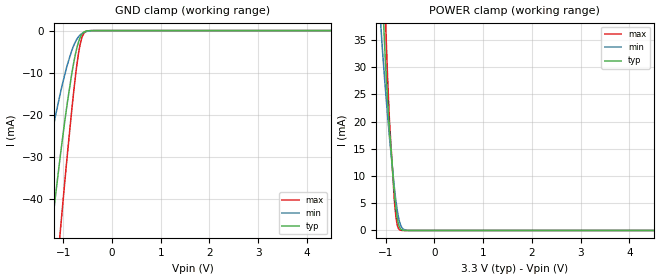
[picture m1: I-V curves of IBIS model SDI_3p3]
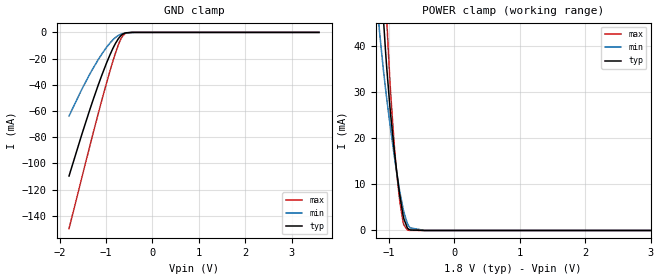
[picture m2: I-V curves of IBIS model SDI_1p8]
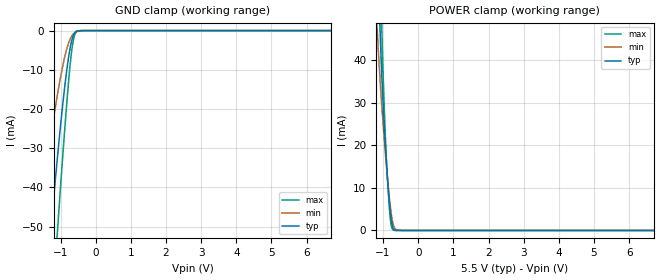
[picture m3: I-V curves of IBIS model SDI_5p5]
|Texas Instruments Incorporated
| 12-Bit Analog Monitor and Control Solution with
| Multichannel ADC, Bipolar DACs adn Temperature Sensors
| Marketing part#   Digital Voltage Range   Package-type   #pins
| AMC7832   1.8V - 5.5V   PQFP   64
[IBIS Ver]   4.1
[File name]   amc7832.ibs
[File Rev]   1.0
[Date]   07/17/2013
[Source]
| Texas Instruments Incorporated.
| Analog-eLab Design Center, HPA
| 12500 TI Blvd
| Dallas, TX -75243
[Notes]   Revision History:
| Rev 1.0: 07/17/2013
| - Initial version of the model
| - Model generated from simulations in TISPICE
| - C_comp although listed in numerical order of value are
|   obtained from varying PVT conditions. For PVT conditions for
|   each specific value refer the buffer description under
|   respective [Model]. IBIS model user is responsible for using
|   appropriate C_comp to simulate for Signal Integrity.
| - Warnings regarding combined Non-monotonicity of various models have been
|   reviewd and considered minor and can be ignored.
| - Model names with a trailing _1p8 contains the model for
|   1.8V operation.Model names with a trailing _3p3 contains the model
|   for 3.3V operation.Model names with a trailing _5p5 contains the model
|   for 5.5V operation.
| - Please note GPIO model is broken into two models depending on its mode
|   of operation (output or input).
[Disclaimer]
| This model is designed as an aid for customers of Texas Instruments.
| TI and its licensors and suppliers make no warranties, either expressed
| or implied, with respect to this  model, including the warranties of
| merchantability or fitness for a particular purpose. The model is
| provided solely on an "as is" basis. The entire risk as to its quality
| and performance is with the customer.
[Copyright]
 (C) Copyright 2013 Texas Instruments Incorporated.All rights reserved.
|   Device
[Component]   TPS51219
[Manufacturer]   TI
[Package]
| PQFP   64
|   typ   min   max
R_pkg   0.116   0.060   0.158
L_pkg   3.087nH   2.446nH   3.790nH
C_pkg   0.477pF   0.441pF   0.609pF
[Pin]  signal_name   model_name   R_pin   L_pin   C_pin
1   DGND   GND   0.07464   2.98837nH   0.48958pF
2   DVDD   POWER   0.13169   3.27499nH   0.48108pF
3   IOVDD   POWER   0.12816   3.19692nH   0.47536pF
4   RESETB   SDI   0.12615   3.14632nH   0.4667pF
5   SDO   SDO   0.12893   3.19318nH   0.46127pF
6   SDI   SDI   0.12666   3.13713nH   0.45672pF
7   SCLK   SDI   0.12544   3.10425nH   0.45279pF
8   CSB   SDI   0.12462   3.08462nH   0.44445pF
9   GPIO0/ALARMINB   GPIO   0.12195   3.03196nH   0.44282pF
10   GPIO1/ALARMOUTB   GPIO   0.12154   3.02759nH   0.45119pF
11   GPIO2/ADCTRIGB   GPIO   0.12196   3.04505nH   0.45655pF
12   GPIO3/DAVB   GPIO   0.12318   3.07964nH   0.46318pF
13   GPIO4   GPIO   0.12516   3.12641nH   0.47241pF
14   GPIO5   GPIO   0.12831   3.19935nH   0.47997pF
15   GPIO6   GPIO   0.13267   3.29462nH   0.48661pF
16   GPIO7   GPIO   0.13863   3.43954nH   0.44655pF
17   AVEE   GND   0.07231   2.94556nH   0.4856pF
18   DAC_A11   NC   0.13114   3.27314nH   0.48478pF
19   DAC_A10   NC   0.12565   3.15687nH   0.47686pF
20   AVSS_A   NC   0.06539   2.59229nH   0.51673pF
21   VRANGE_A   NC   0.12005   3.02694nH   0.45909pF
22   DAC_A9   NC   0.11967   3.00768nH   0.45569pF
23   AGND1   GND   0.06348   2.50448nH   0.4998pF
24   DAC_A8   NC   0.11877   2.97614nH   0.44498pF
25   AVCC_AB   POWER   0.06352   2.44605nH   0.49873pF
26   VRANGE_B   NC   0.1175   2.95523nH   0.4486pF
27   DAC_B7   NC   0.12033   3.02069nH   0.45459pF
28   AVSS_B   GND   0.06484   2.56764nH   0.51127pF
29   DAC_B6   NC   0.12376   3.1084nH   0.4693pF
30   REF_OUT1   NC   0.12489   3.14114nH   0.47142pF
31   AVDD1   POWER   0.12943   3.23893nH   0.48258pF
32   REF_CMP   NC   0.07299   2.86238nH   0.49781pF
33   AGND2   GND   0.06024   3.09923nH   0.58549pF
34   AVDD2   POWER   0.08563   3.23091nH   0.60933pF
35   ADC_11   NC   0.15758   3.7897nH   0.52144pF
36   ADC_10   NC   0.14845   3.5965nH   0.5063pF
37   ADC_9   NC   0.14092   3.43726nH   0.49064pF
38   ADC_8   NC   0.13472   3.30228nH   0.47781pF
39   ADC_7   NC   0.12993   3.19697nH   0.46698pF
40   ADC_6   NC   0.12655   3.12518nH   0.455pF
41   LV_ADC16   NC   0.12409   3.07578nH   0.44888pF
42   LV_ADC15   NC   0.1236   3.07045nH   0.45215pF
43   LV_ADC14   NC   0.12381   3.08372nH   0.4563pF
44   LV_ADC13   NC   0.12473   3.11302nH   0.46145pF
45   LV_ADC_12   NC   0.1263   3.15208nH   0.46839pF
46   ADC_5   NC   0.12888   3.2135nH   0.47766pF
47   ADC_4   NC   0.13439   3.32975nH   0.48914pF
48   ADC_3   NC   0.14231   3.51158nH   0.45064pF
49   ADC_2   NC   0.13353   3.33493nH   0.44139pF
50   ADC_1   NC   0.12597   3.15979nH   0.47985pF
51   ADC_0   NC   0.12099   3.05316nH   0.46759pF
52   DAC_C0   NC   0.12205   3.06323nH   0.46543pF
53   AVSS_C   GND   0.06421   2.5389nH   0.50917pF
54   DAC_C1   NC   0.11943   2.99201nH   0.45501pF
55   VRANGE_C   NC   0.11829   2.9599nH   0.4497pF
56   REF_OUT2   NC   0.11893   2.96848nH   0.44539pF
57   AVCC_CD   POWER   0.06422   2.46561nH   0.5006pF
58   DAC_D2   NC   0.12085   3.01039nH   0.45506pF
59   AGND3   GND   0.06535   2.574nH   0.51014pF
60   DAC_D3   NC   0.12454   3.10478nH   0.46658pF
61   VRANGE_D   NC   0.12732   3.16823nH   0.47473pF
62   AVSS_D   GND   0.06959   2.7448nH   0.53356pF
63   DAC_D4   NC   0.13598   3.35887nH   0.49213pF
64   DAC_D5   NC   0.14445   3.55251nH   0.45417pF
|   Model Selectors
[Model Selector]  SDI
SDI_3p3   input buffer with 3.3V operation
SDI_1p8   input buffer with 1.8V operation
SDI_5p5   input buffer with 5.5V operation
[Model Selector]  SDO
SDO_3p3   output buffer with 3.3V operation
SDO_1p8   output buffer with 1.8V operation
SDO_5p5   output buffer with 5.5V operation
[Model Selector]  GPIO
GPIO_OUT_3p3   ouput mode with 3.3V operation
GPIO_OUT_1p8   ouput mode with 1.8V operation
GPIO_OUT_5p5   ouput mode with 5.5V operation
GPIO_IN_3p3   input mode with 3.3V operation
GPIO_IN_1p8   input mode with 1.8V operation
GPIO_IN_5p5   input mode with 5.5V operation
| Models and submodels in the file (12): SDI_3p3 (Input), SDI_1p8 (Input), SDI_5p5 (Input), SDO_5p5 (Output), SDO_3p3 (Output), SDO_1p8 (Output), GPIO_OUT_5p5 (Output), GPIO_OUT_3p3 (Output), GPIO_OUT_1p8 (Output), GPIO_IN_5p5 (Input), GPIO_IN_3p3 (Input), GPIO_IN_1p8 (Input)
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|   Model
[Model]   SDI_3p3
Model_type   Input
Vinl = 0.99
Vinh = 2.31
|   typ   min   max
C_comp   1pF   1pF   1pF
[Voltage Range]   3.3   3.29   3.31
[Temperature Range]   27   125   -40
[Power Clamp Reference]   3.3   3.29   3.31
[GND Clamp Reference]   -0   -0   -0
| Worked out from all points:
|   GND clamp passes 1 mA (typ) near -0.62 V on its own axis
|   POWER clamp passes 1 mA (typ) near -0.73 V on its own axis
[GND Clamp]
|   Voltage   I(typ)   I(min)   I(max)
-3.3V     -293.4mA   -195.7mA   -362.8mA
-1.607V   -87.33mA   -49.37mA   -122.6mA
-1.498V   -75.05mA   -41.65mA   -107.3mA
-1.241V   -47.39mA   -24.95mA   -71.62mA
-1.063V   -29.88mA   -14.98mA   -47.85mA
-914.1mV  -16.91mA   -8.021mA   -29.15mA
-825mV    -10.21mA   -4.72mA    -18.75mA
-735.9mV  -4.854mA   -2.34mA    -9.493mA
-646.8mV  -1.481mA   -966.8uA   -2.922mA
-597.3mV  -576.8uA   -553.5uA   -1.078mA
-547.8mV  -186.8uA   -301.2uA   -307.2uA
6.59V     0A         0A         0A
[POWER Clamp]
|   Voltage   I(typ)   I(min)   I(max)
-3.3V     807.6mA    663.4mA    932mA
-1.122V   56.01mA    40.38mA    75.28mA
-1.063V   41.86mA    32.46mA    55.66mA
-1.023V   33.91mA    27.73mA    43.65mA
-1.003V   30.38mA    25.49mA    38.12mA
-924mV    18.55mA    17.08mA    20.11mA
-825mV    7.046mA    7.968mA    5.687mA
-765.6mV  2.369mA    3.793mA    1.093mA
-706.2mV  402.6uA    1.259mA    79.14uA
-636.9mV  31.36uA    230.3uA    2.758uA
-518.1mV  231.3nA    8.259uA    0A
6.59V     0A         0A         0A
|   Model
[Model]   SDI_1p8
Model_type   Input
Vinl = 0.45
Vinh = 1.26
|   typ   min   max
C_comp   1pF   1pF   1pF
[Voltage Range]   1.8   1.79   1.81
[Temperature Range]   27   125   -40
[Power Clamp Reference]   1.8   1.79   1.81
[GND Clamp Reference]   -0   -0   -0
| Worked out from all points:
|   GND clamp passes 1 mA (typ) near -0.62 V on its own axis
|   POWER clamp passes 1 mA (typ) near -0.73 V on its own axis
[GND Clamp]
|   Voltage   I(typ)   I(min)   I(max)
-1.8V     -109.7mA   -63.85mA   -149.9mA
-1.525V   -78mA      -43.49mA   -111mA
-1.363V   -60.2mA    -32.55mA   -88.36mA
-1.168V   -40.05mA   -20.71mA   -61.81mA
-990mV    -23.31mA   -11.39mA   -38.54mA
-855mV    -12.35mA   -5.739mA   -22.16mA
-736.2mV  -4.869mA   -2.347mA   -9.521mA
-682.2mV  -2.547mA   -1.401mA   -5.068mA
-639mV    -1.295mA   -888.1uA   -2.543mA
-595.8mV  -558.8uA   -543.9uA   -1.041mA
-428.4mV  -7.854uA   -47.81uA   -7.097uA
3.595V    0A         0A         0A
[POWER Clamp]
|   Voltage   I(typ)   I(min)   I(max)
-1.8V     276.3mA    209.7mA    333mA
-1.141V   61.07mA    43.23mA    81.91mA
-1.076V   44.93mA    34.19mA    60.07mA
-1.028V   34.81mA    28.29mA    45.05mA
-968.4mV  24.8mA     21.69mA    29.34mA
-914.4mV  17.29mA    16.12mA    18.38mA
-876.6mV  12.63mA    12.48mA    12.33mA
-828mV    7.34mA     8.212mA    6.019mA
-779.4mV  3.229mA    4.636mA    1.778mA
-714.6mV  536.5uA    1.507mA    118uA
-450mV    0A         1.128uA    0A
3.595V    0A         0A         0A
|   Model
[Model]   SDI_5p5
Model_type   Input
Vinl = 1.65
Vinh = 3.85
|   typ   min   max
C_comp   1pF   1pF   1pF
[Voltage Range]   5.5   5.49   5.51
[Temperature Range]   27   125   -40
[Power Clamp Reference]   5.5   5.49   5.51
[GND Clamp Reference]   -0   -0   -0
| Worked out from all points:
|   GND clamp passes 1 mA (typ) near -0.62 V on its own axis
|   POWER clamp passes 1 mA (typ) near -0.73 V on its own axis
[GND Clamp]
|   Voltage   I(typ)   I(min)   I(max)
-5.5V     -568.4mA   -435.6mA   -672.5mA
-1.623V   -89.08mA   -50.49mA   -124.8mA
-1.375V   -61.53mA   -33.35mA   -90.08mA
-1.26V    -49.31mA   -26.08mA   -74.17mA
-1.095V   -32.89mA   -16.65mA   -52.02mA
-896.5mV  -15.51mA   -7.307mA   -27.03mA
-797.5mV  -8.388mA   -3.877mA   -15.73mA
-731.5mV  -4.635mA   -2.25mA    -9.087mA
-649mV    -1.536mA   -990uA     -3.035mA
-599.5mV  -604.2uA   -567.9uA   -1.133mA
-533.5mV  -131.6uA   -249.6uA   -205.7uA
10.98V    0A         0A         0A
[POWER Clamp]
|   Voltage   I(typ)   I(min)   I(max)
-5.5V     1.598A     1.344A     1.82A
-1.21V    80.56mA    55mA       106.4mA
-1.161V   66.34mA    46.28mA    88.68mA
-1.111V   53.21mA    38.81mA    71.54mA
-1.078V   45.29mA    34.4mA     60.59mA
-1.045V   38.17mA    30.32mA    50.19mA
-1.028V   34.94mA    28.37mA    45.25mA
-946mV    21.55mA    19.33mA    24.41mA
-863.5mV  11.12mA    11.28mA    10.47mA
-781mV    3.338mA    4.739mA    1.874mA
-682mV    169.4uA    722.7uA    24.67uA
10.98V    0A         0A         0A
